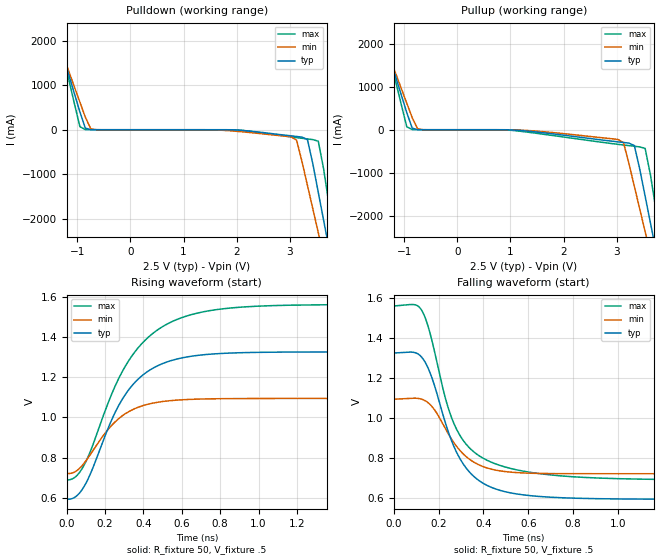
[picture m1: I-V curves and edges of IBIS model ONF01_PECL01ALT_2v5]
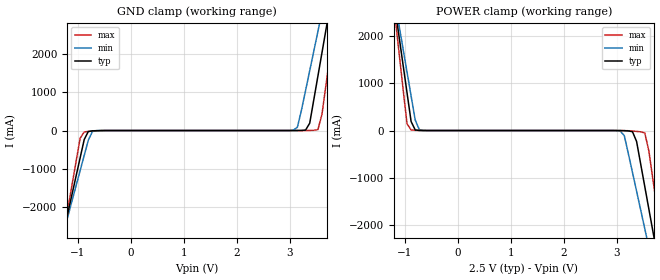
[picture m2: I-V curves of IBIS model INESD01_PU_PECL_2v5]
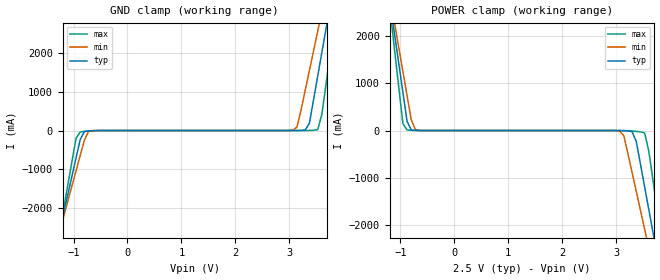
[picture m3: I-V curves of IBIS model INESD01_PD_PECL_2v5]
|   This file is an IBIS representation of the   |
|   Integrated Devices Technology, Inc.   |
|   ICS85311I   |
|   1 o 2 Differentail to ECL/LVPECL Fanout Buffer   |
[IBIS Ver]   4.1
[File name]   85311i.ibs
[File Rev]   1.0
[Date]   23 Dec 2008 | Last modified
|   Aug 14 2001 | Generated
[Source]   Originated at Integrated Devices Technology, Inc.
[Disclaimer]
IDT hereby grants the user of this IBIS model a non-exclusive,
nontransferable license to use this IBIS model under the following terms.
Before using this IBIS model, the user should read this license.
If the user does not accept these terms,  the IBIS model should be
returned to IDT within 30 days.
   The user is granted this license only to use the IBIS model and
is not granted rights to sell, load, rent, lease or license the IBIS
model in whole or in part, or in modified form to anyone other than
user. User may modify the IBIS model to suit its specific
applications but rights to derivative works and such modifications
shall belong to IDT.
   This IBIS model is provided on an "AS IS" basis and IDT makes
absolutely no warranty with respect to the information contained
herein. IDT DISCLAIMS AND CUSTOMER WAIVES ALL WARRANTIES, EXPRESS
OR IMPLIED, INCLUDING WARRANTIES OF MERCHANTABILITY OR FITNESS FOR
A PARTICULAR PURPOSE. The entire risk as to quality and performance
is with the Customer. ACCORDINGLY, IN NO EVENT SHALL THE COMPANY BE
LIABLE FOR ANY DAMAGES, WHETHER IN CONTRACT OR TORT,INCLUDING ANY
LOST PROFITS OR OTHER INCIDENTAL, CONSEQUENTIAL, EXEMPLARY, OR
PUNITIVE DAMAGES ARISING OUT OF THE USE OR APPLICATION OF THE IBIS
model provided in this package. Further, IDT reserves the right to
make changes without notice to any product herein to improve
reliability, function, or design. IDT does not convey any license
under patent rights or any other intellectual property rights,
including those of third parties.
   IDT is not obligated to provide maintenance or support
for the licensed IBIS model.
[Copyright]   Copyright 2004 byIntegrated Devices Technology, Inc.
[Component]   ICS85311
[Manufacturer] Integrated Devices Technology, Inc.
[Package]
|SOIC 8 Lead
|   typ   min   max
R_pkg   57.05m   55.5m   58.6m
L_pkg   1.769nH   1.570nH   1.968nH
C_pkg   0.269pF   0.252pF   0.286pF
[Pin]   signal_name   model_name   R_pin   L_pin   C_pin
1   Q0   ONF01_PECL01ALT   58.6m   1.968n   0.286p
2   nQ0   ONF01_PECL01ALT   55.5m   1.570n   0.252p
3   Q1   ONF01_PECL01ALT   55.5m   1.570n   0.252p
4   nQ1   ONF01_PECL01ALT   56.6m   1.968n   0.286p
5   VEE   GND   58.6m   1.968n   0.286p
6   nCLK   INESD01_PU_PECL   55.5m   1.570n   0.252p
7   CLK   INESD01_PD_PECL   55.5m   1.570n   0.252p
8   VCC   POWER   56.6m   1.968n   0.286p
[Diff Pin]  inv_pin  vdiff tdelay_typ tdelay_min  tdelay_max
|Input
7   6   0.15   0   0   0
|Output
1   2   NA   0   0   0
3   4   NA   0   0   0
[Model Selector] ONF01_PECL01ALT
ONF01_PECL01ALT_2v5  Buffer selection for 2v5
ONF01_PECL01ALT_3v3  Buffer selection for 3v3
[Model Selector] INESD01_PU_PECL
INESD01_PU_PECL_2v5  Buffer selection for 2v5
INESD01_PU_PECL_3v3  Buffer selection for 3v3
[Model Selector] INESD01_PD_PECL
INESD01_PD_PECL_2v5  Buffer selection for 2v5
INESD01_PD_PECL_3v3  Buffer selection for 3v3
| Models and submodels in the file (6): ONF01_PECL01ALT_2v5 (Output_ECL), INESD01_PU_PECL_2v5 (Input), INESD01_PD_PECL_2v5 (Input), ONF01_PECL01ALT_3v3 (Output_ECL), INESD01_PU_PECL_3v3 (Input), INESD01_PD_PECL_3v3 (Input)
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[Model] ONF01_PECL01ALT_2v5
Model_type  Output_ECL
Polarity   Non-Inverting
Vmeas = .975
Rref = 50
Cref = 0
Vref = .5
|Variable  typ   min   max
C_comp   2p   1.5p   2.5p
[Voltage Range]   2.5   2.375   2.625
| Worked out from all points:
|   rising waveform, R_fixture 50, V_fixture .5: 20-80 % time 228ps typ, 199ps min, 276ps max; typ from 0.592 V to 1.33 V
|   falling waveform, R_fixture 50, V_fixture .5: 20-80 % time 153ps typ, 140ps min, 156ps max; typ from 1.33 V to 0.592 V
| Open source, no load
|  Voltage   I(typ)   I(min)   I(max)
[Pullup]
-3.3V     9.786A     8.425A     12.06A
-1.463V   2.432A     2.308A     2.661A
-952.6mV  398mA      618.5mA    68.87mA
-850.5mV  36.63mA    281.6mA    4.032mA
-646.4mV  229.3uA    964.8uA    177.5uA
3.028V    -282.4mA   -226.8mA   -340.1mA
3.13V     -296.5mA   -301.7mA   -355.4mA
3.334V    -367.3mA   -1.316A    -385.1mA
3.538V    -1.551A    -2.377A    -435.3mA
3.64V     -2.187A    -2.908A    -1.066A
3.844V    -3.46A     -3.969A    -2.688A
6.6V      -20.66A    -18.32A    -24.61A
[Pulldown]
-3.3V     9.786A     8.425A     12.06A
-1.463V   2.432A     2.308A     2.661A
-1.361V   2.024A     1.97A      2.139A
-952.6mV  398mA      618.5mA    68.87mA
-850.5mV  36.63mA    281.6mA    4.032mA
3.028V    -137.6mA   -160.7mA   -160.7mA
3.13V     -151.4mA   -235.1mA   -176.3mA
3.334V    -221.9mA   -1.249A    -206.7mA
3.538V    -1.406A    -2.31A     -257.4mA
3.64V     -2.042A    -2.84A     -888.8mA
3.844V    -3.314A    -3.9A      -2.51A
6.6V      -20.58A    -18.26A    -24.54A
[Ramp]
|   typ   min   max
dV/dt_r   0.586/0.368n   0.299/0.313n   0.698/0.446n
dV/dt_f   0.586/0.258n   0.299/0.226n   0.698/0.290n
R_load =   50.0000
[Rising Waveform]
R_fixture = 50
V_fixture = .5   | VCC_typ - 2V
V_fixture_max = 0.625   | VCC_max - 2V
V_fixture_min = 0.375   | VCC_min - 2V
C_fixture = 0.0p
| Time   typ   min   max
0s        592.5mV    720.8mV    689.3mV
46.2ps    605.5mV    731.1mV    704.8mV
92.4ps    659.4mV    774.5mV    766.4mV
241.5ps   1.003V     967.6mV    1.133V
323.4ps   1.138V     1.029V     1.283V
426.3ps   1.231V     1.066V     1.4V
552.3ps   1.285V     1.084V     1.478V
711.9ps   1.312V     1.092V     1.525V
940.8ps   1.323V     1.094V     1.551V
1.999ns   1.326V     1.094V     1.562V
[Falling Waveform]
R_fixture = 50
V_fixture = .5   | VCC_typ - 2V
V_fixture_max = 0.625   | VCC_max - 2V
V_fixture_min = 0.375   | VCC_min - 2V
C_fixture = 0.0p
0s        1.326V     1.094V     1.562V
92.4ps    1.328V     1.099V     1.568V
123.9ps   1.306V     1.095V     1.541V
168ps     1.209V     1.061V     1.4V
231ps     973.8mV    945.4mV    1.097V
277.2ps   835.9mV    862.7mV    951mV
348.6ps   716.5mV    784.8mV    838.7mV
447.3ps   647.2mV    740.6mV    773mV
865.2ps   596.5mV    720.8mV    701.4mV
1.999ns   592.4mV    720.7mV    689.3mV
[Model] INESD01_PU_PECL_2v5
Model_type  Input
Polarity   Non-Inverting
Vinl = 0.9
Vinh = 1.6V
|   typ   min   max
C_comp   2pF   1.5pF   2.5pF
|   typ   min   max
[Voltage range]  2.5V   2.375V   2.625V
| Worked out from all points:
|   GND clamp passes 1 mA (typ) near -0.54 V on its own axis
|   POWER clamp passes 1 mA (typ) near -0.67 V on its own axis
[GND_clamp]
|Voltage   I(typ)   I(min)   I(max)
-2.5V     -10.33A    -9.044A    -12.47A
-1.263V   -2.632A    -2.639A    -2.655A
-953.6mV  -711.7mA   -1.044A    -200.4mA
-876.3mV  -232.8mA   -646mA     -36.9mA
-644.3mV  -3.744mA   -3.442mA   -8.163mA
3.067V    100.7uA    7.657mA    8.292uA
3.144V    453.6uA    86.78mA    24.43uA
3.376V    191.1mA    1.558A     2.391mA
3.531V    1.418A     2.581A     23.29mA
3.686V    2.649A     3.605A     1.215A
3.84V     3.882A     4.631A     2.791A
5V        13.16A     12.34A     14.65A
[POWER_clamp]
|Voltage   I(typ)   I(min)   I(max)
-2.5V     13.16A     11.51A     15.93A
-1.186V   2.649A     2.777A     2.489A
-1.108V   2.034A     2.265A     1.701A
-953.6mV  804mA      1.243A     144.3mA
-876.3mV  191.1mA    733mA      11.81mA
-644.3mV  453.6uA    1.831mA    349.6uA
3.067V    -1.275mA   -11.3mA    -266.4uA
3.299V    -24.55mA   -891.1mA   -10.77mA
3.531V    -1.191A    -2.086A    -51.94mA
3.686V    -2.151A    -2.885A    -1.049A
3.84V     -3.112A    -3.684A    -2.276A
5V        -10.33A    -9.692A    -11.48A
[Model] INESD01_PD_PECL_2v5
Model_type  Input
Polarity   Non-Inverting
Vinl = 0.9
Vinh = 1.6V
|   typ   min   max
C_comp   2pF   1.5pF   2.5pF
|   typ   min   max
[Voltage range]  2.5V   2.375V   2.625V
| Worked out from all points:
|   GND clamp passes 1 mA (typ) near -0.55 V on its own axis
|   POWER clamp passes 1 mA (typ) near -0.67 V on its own axis
[GND_clamp]
|Voltage   I(typ)   I(min)   I(max)
-2.5V     -10.33A    -9.044A    -12.47A
-1.263V   -2.632A    -2.639A    -2.655A
-953.6mV  -711.7mA   -1.044A    -200.4mA
-876.3mV  -232.7mA   -645.9mA   -36.86mA
-644.3mV  -3.696mA   -3.384mA   -8.124mA
3.067V    149.4uA    7.715mA    47.92uA
3.144V    502.3uA    86.83mA    64.06uA
3.376V    191.2mA    1.558A     2.431mA
3.531V    1.419A     2.581A     23.33mA
3.686V    2.649A     3.605A     1.215A
3.84V     3.882A     4.631A     2.791A
5V        13.16A     12.34A     14.65A
[POWER_clamp]
|Voltage   I(typ)   I(min)   I(max)
-2.5V     13.16A     11.51A     15.93A
-1.186V   2.649A     2.777A     2.489A
-1.108V   2.034A     2.265A     1.701A
-953.6mV  804mA      1.243A     144.3mA
-876.3mV  191.2mA    733.1mA    11.85mA
-644.3mV  502.3uA    1.889mA    389.3uA
3.067V    -1.226mA   -11.24mA   -226.8uA
3.299V    -24.5mA    -891.1mA   -10.73mA
3.531V    -1.191A    -2.086A    -51.9mA
3.686V    -2.151A    -2.885A    -1.049A
3.84V     -3.112A    -3.684A    -2.276A
5V        -10.33A    -9.692A    -11.48A
